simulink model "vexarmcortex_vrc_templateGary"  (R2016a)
settings: Solver=FixedStepDiscrete  StartTime=0.0  StopTime=inf  RelTol=1e-3
libraries: vexarmcortexlib x7

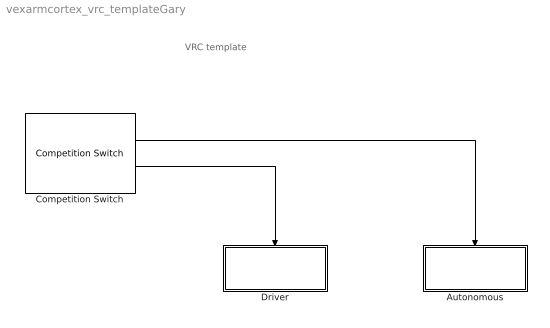
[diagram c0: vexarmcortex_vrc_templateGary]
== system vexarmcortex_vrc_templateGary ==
  note: VRC template
  Autonomous : Subsystem  TreatAsAtomicUnit=on
  Competition Switch : vexarmcortexlib/Competition Switch  SampleTime=0.2
  Driver : Subsystem  TreatAsAtomicUnit=on
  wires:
  Competition Switch/2 -> Driver/Enable
  Competition Switch/1 -> Autonomous/Enable

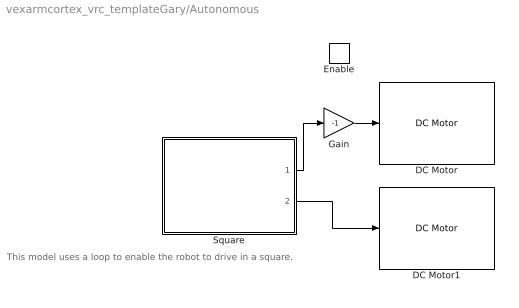
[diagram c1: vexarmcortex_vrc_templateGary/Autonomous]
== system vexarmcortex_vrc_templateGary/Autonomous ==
  note: This model uses a loop to enable the robot to drive in a square.
  Enable : EnablePort
  DC Motor : vexarmcortexlib/DC Motor  motor=3  scaleFactor=1/13.5  SimulationOut=on
  DC Motor1 : vexarmcortexlib/DC Motor  motor=7  scaleFactor=1/13.5  SimulationOut=on
  Gain : Gain  Gain=-1
  Square : Stateflow chart  TreatAsAtomicUnit=on
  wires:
  Gain/1 -> DC Motor/1
  Square/1(speedL) -> Gain/1
  Square/2(speedR) -> DC Motor1/1

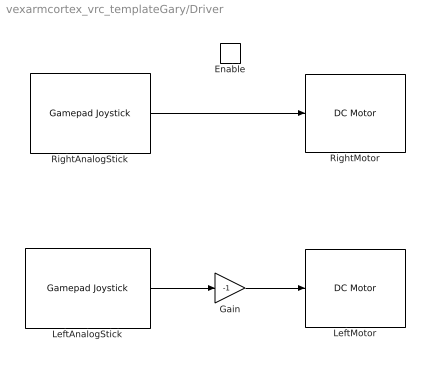
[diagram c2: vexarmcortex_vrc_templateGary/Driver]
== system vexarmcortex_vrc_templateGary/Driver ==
  Enable : EnablePort
  Gain : Gain  Gain=-1
  LeftAnalogStick : vexarmcortexlib/Gamepad Joystick  joystick=1  chan=3  SimulationIn=on
  LeftMotor : vexarmcortexlib/DC Motor  motor=3  scaleFactor=1/13.5  SimulationOut=on
  RightAnalogStick : vexarmcortexlib/Gamepad Joystick  joystick=1  chan=2  SimulationIn=on
  RightMotor : vexarmcortexlib/DC Motor  motor=7  scaleFactor=1/13.5  SimulationOut=on
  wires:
  RightAnalogStick/1 -> RightMotor/1
  LeftAnalogStick/1 -> Gain/1
  Gain/1 -> LeftMotor/1

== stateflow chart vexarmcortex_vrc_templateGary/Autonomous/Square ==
  state Halt
    during:
    speedL = 0;
    speedR = 0;
  state TurnRight
    during:
    speedL = 42;
    speedR = -42;
  state Forward
    during:
    speedL = 100;
    speedR = 100;
    entry:
    count = count +1;
  state FullStop
    during:
    speedL = 0;
    speedR = 0;
  state Note that there is a counter which [group]
    increases the index every time the
    loop enters the State called Forward
  TurnRight -> Halt : after(1,sec)
  Halt -> Forward : after(1,sec)
  Forward -> TurnRight : after(4,sec)
  Forward -> FullStop : [count>4]
  (default) -> Forward : {count = 0;}
  data: speedL output; speedR output; count local
